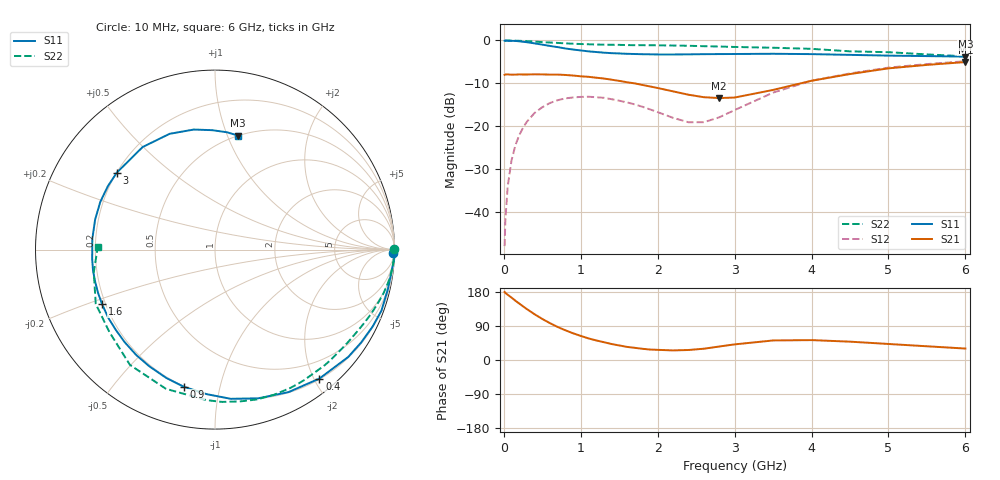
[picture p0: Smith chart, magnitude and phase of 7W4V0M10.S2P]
! Infineon Technologies  Discrete & RF Semiconductors
! BFS17W
! Si NPN RF Bipolar Junction Transistor in SOT323
! VCE = 4 V  IC = 0.1 mA
! Common Emitter S-Parameters:  August  1999
# GHz  S  MA  R  50
!  f  S11  S21  S12  S22
! GHz  MAG  ANG  MAG  ANG  MAG  ANG  MAG  ANG
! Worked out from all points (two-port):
!   36 points, 10 MHz to 6 GHz, reference 50 ohm
!   highest |S21| = -5.04 dB at 6 GHz (marker M1); lowest = -13.4 dB at 2.8 GHz (marker M2)
!   |S21| within 3 dB of the highest: start of sweep to 788.7 MHz; 4.434 GHz to end of sweep
!   lowest |S11| = -3.8 dB at 6 GHz (marker M3), VSWR 4.68, Z = 25 + j54.7 ohm
!   |S11| at or under -10 dB: nowhere
!   |S22| runs from -3.7 to 0.0 dB; largest |S21 - S12| = 0.4
!   S11 on the Smith chart (normalised r, x): 10 MHz: 25, -88; 400 MHz: 0.21, -2.08; 900 MHz: 0.20, -0.78; 1.6 GHz: 0.19, -0.22; 3 GHz: 0.20, +0.33; 6 GHz: 0.50, +1.09
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0.01  0.9941 -1.2  0.397 179.4  0.004 87.7  0.9999 0.1
0.02  0.9999 -2.9  0.401 176.9  0.0081 87.6  0.9897 -0.7
0.05  0.9919 -6.6  0.402 172.3  0.0198 87.1  0.9986 -1.9
0.1  0.9882 -12.9  0.399 164.7  0.04 81.9  0.9966 -3.8
0.15  0.9878 -20.2  0.4 156.5  0.0599 77.0  0.9937 -5.7
0.2  0.9771 -26.1  0.402 149.0  0.0787 73.4  0.9902 -7.4
0.4  0.9244 -51.0  0.403 120.6  0.143 57.3  0.9702 -14.4
0.6  0.8628 -73.8  0.4 97.2  0.1867 44.0  0.9463 -20.6
0.9  0.7835 -102.9  0.39 70.5  0.2165 28.0  0.9158 -29.4
1.1  0.746 -119.5  0.377 57.0  0.2208 20.0  0.9026 -35.0
1.3  0.7205 -134.4  0.36 47.0  0.2146 13.4  0.8925 -40.8
1.6  0.6987 -154.1  0.326 34.6  0.1898 6.7  0.8834 -49.4
2.2  0.6861 175.0  0.255 25.3  0.1253 13.3  0.8731 -67.9
2.6  0.6922 157.4  0.218 29.8  0.1114 40.8  0.8571 -80.8
2.8  0.6937 149.4  0.213 35.6  0.127 54.0  0.8496 -87.3
3  0.6951 141.9  0.216 41.2  0.1543 62.7  0.84 -93.3
3.5  0.6994 125.2  0.265 51.6  0.2466 67.5  0.8224 -109.4
4  0.6929 111.4  0.339 52.5  0.3399 61.9  0.7982 -126.4
4.5  0.6792 100.0  0.406 48.4  0.4129 54.0  0.7466 -142.0
5  0.6655 91.3  0.473 42.3  0.4825 46.2  0.73 -155.5
5.5  0.6571 84.2  0.519 36.2  0.5306 38.8  0.6873 -169.4
6  0.648 78.5  0.56 30.2  0.5729 32.1  0.6531 178.7
